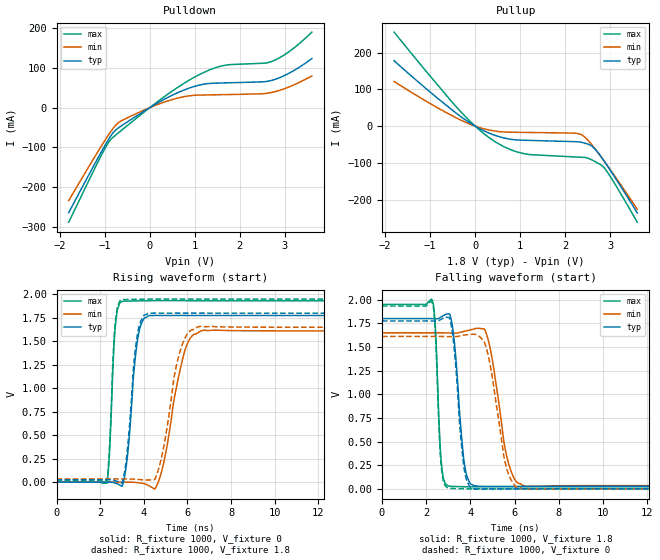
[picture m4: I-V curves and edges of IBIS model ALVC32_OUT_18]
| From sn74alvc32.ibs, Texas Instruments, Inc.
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[Model]   ALVC32_OUT_18
Model_type  Output
Vref =   0
Rref =   1000
Cref =   30p
Vmeas =   0.9
| variable   typ   min   max
C_comp   8.44pF   5.76pF   11.61pF
| C_pullup   8.56pF   6.36pF   9.74pF
| C_pulldown   8.32pF   5.76pF   11.61pF
[Temperature Range]   40   100   -40
| Ambient temperature   25   85   -40
[Voltage range]   1.8   1.65   1.95
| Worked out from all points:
|   slope of the pulldown table from 0 to 0.27 V, typ, clamps not added: 15.1 ohm
|   slope of the pullup table from 0 to 0.27 V, typ, clamps not added: 15.9 ohm
|   rising waveform, R_fixture 1000, V_fixture 0: 20-80 % time 373ps typ, 742ps min, 215ps max; typ from 0 V to 1.77 V
|   falling waveform, R_fixture 1000, V_fixture 1.8: 20-80 % time 351ps typ, 614ps min, 198ps max; typ from 1.8 V to 0.026 V
|   rising waveform, R_fixture 1000, V_fixture 1.8: 20-80 % time 370ps typ, 688ps min, 212ps max; typ from 0.026 V to 1.8 V
|   falling waveform, R_fixture 1000, V_fixture 0: 20-80 % time 351ps typ, 622ps min, 197ps max; typ from 1.77 V to 0 V
[Pulldown]
| ALVC32_OUT_18
|   Voltage   I(typ)   I(min)   I(max)
-1.8V     -264.5mA   -234.1mA   -288.3mA
-1.155V   -127.9mA   -111.4mA   -137.9mA
-915mV    -80.08mA   -68.36mA   -87.27mA
-800mV    -61.37mA   -50.08mA   -73.15mA
-690mV    -50.59mA   -37.38mA   -62.82mA
-210mV    -14.85mA   -10.42mA   -18.81mA
550mV     34.08mA    22.06mA    45.73mA
1.16V     58.24mA    31.77mA    86.5mA
1.675V    62.35mA    32.87mA    106.8mA
2.71V     68.82mA    38.41mA    116.5mA
3.115V    88.05mA    53.24mA    142.8mA
3.6V      123.5mA    79.91mA    190.3mA
[Pullup]
| ALVC32_OUT_18
|   Voltage   I(typ)   I(min)   I(max)
-1.8V     177.9mA    121.4mA    255.7mA
-380mV    31.41mA    20.06mA    47.26mA
40mV      -2.839mA   -1.667mA   -4.509mA
390mV     -22.94mA   -12.43mA   -38.14mA
740mV     -34.79mA   -16.58mA   -61.65mA
1.095V    -38.57mA   -17.2mA    -75.19mA
2.195V    -42.3mA    -19.18mA   -83.81mA
2.365V    -44.23mA   -23.75mA   -84.88mA
2.61V     -56.21mA   -53.66mA   -93.1mA
2.865V    -95.44mA   -95.17mA   -113.5mA
3.105V    -139.7mA   -136.8mA   -157.6mA
3.6V      -236.1mA   -226.1mA   -261.5mA
[Ramp]
| ALVC32_OUT_18
| variable   typ   min   max
dV/dt_r   1.09/3.92E-10   1.01/8.07E-10   1.17/2.40E-10
dV/dt_f   1.09/3.70E-10   1.00/7.26E-10   1.19/2.12E-10
R_load = 1000
[Rising Waveform]
| ALVC32_OUT_18
R_fixture =   1000
C_fixture =   0
L_fixture =   0
V_fixture =   0
V_fixture_min = 0
V_fixture_max = 0
|   Time   V(typ)   V(min)   V(max)
0s        30.49pV    5.701nV    21.71pV
2.32ns    871.2uV    259.6uV    -10.22mV
2.695ns   -10.51mV   700.2uV    1.663V
3.07ns    6.067mV    554uV      1.929V
3.715ns   1.521V     -5.163mV   1.931V
4.275ns   1.776V     -43.06mV   1.933V
4.835ns   1.775V     131.3mV    1.933V
5.895ns   1.776V     1.413V     1.933V
6.72ns    1.776V     1.617V     1.933V
50ns      1.775V     1.611V     1.933V
[Falling Waveform]
| ALVC32_OUT_18
R_fixture =   1000
C_fixture =   0
L_fixture =   0
V_fixture =   1.8
V_fixture_min = 1.65
V_fixture_max = 1.95
|   Time   V(typ)   V(min)   V(max)
0s        1.8V       1.65V      1.95V
2.285ns   1.799V     1.65V      1.988V
2.68ns    1.818V     1.65V      296.7mV
3.02ns    1.85V      1.648V     29.09mV
3.735ns   259.1mV    1.666V     22.24mV
4.19ns    30.47mV    1.692V     21.34mV
4.735ns   25.57mV    1.634V     21.29mV
5.705ns   24.9mV     288.2mV    21.64mV
6.515ns   25.26mV    25.77mV    21.74mV
50ns      25.59mV    33.88mV    21.73mV
[Rising Waveform]
| ALVC32_OUT_18
R_fixture =   1000
C_fixture =   0
L_fixture =   0
V_fixture =   1.8
V_fixture_min = 1.65
V_fixture_max = 1.95
|   Time   V(typ)   V(min)   V(max)
0s        25.59mV    33.88mV    21.73mV
2.32ns    26.3mV     34.13mV    18.35mV
2.685ns   16.14mV    34.42mV    1.68V
3.055ns   34.44mV    34.08mV    1.946V
3.695ns   1.555V     29.91mV    1.948V
4.255ns   1.802V     23.16mV    1.95V
4.77ns    1.8V       222.3mV    1.95V
5.705ns   1.8V       1.428V     1.95V
6.575ns   1.8V       1.659V     1.95V
50ns      1.8V       1.65V      1.95V
[Falling Waveform]
| ALVC32_OUT_18
R_fixture =   1000
C_fixture =   0
L_fixture =   0
V_fixture =   0
V_fixture_min = 0
V_fixture_max = 0
|   Time   V(typ)   V(min)   V(max)
0s        1.775V     1.611V     1.933V
2.275ns   1.774V     1.611V     1.97V
2.675ns   1.792V     1.611V     261.7mV
3.005ns   1.812V     1.61V      8.547mV
3.72ns    212.4mV    1.625V     434uV
4.215ns   -3.742mV   1.634V     -421uV
4.79ns    -712.5uV   1.429V     -403.1uV
5.685ns   -482.1uV   183.7mV    -97.05uV
6.4ns     -274uV     -3.674mV   -3.254uV
50ns      30.56pV    5.527nV    21.23pV
